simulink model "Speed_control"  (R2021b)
settings: Solver=ode1  StartTime=0.0  StopTime=inf  FixedStep=0.002  RelTol=1e-3  EnableMultiTasking=on
undefined symbols (not defined in the file or in its folder): HIL, qc_get_step_size
libraries: quarc_library x3

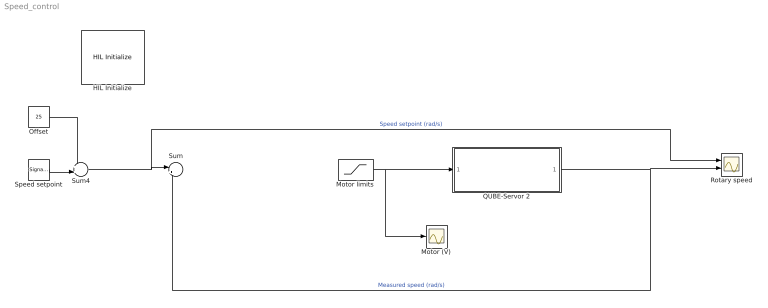
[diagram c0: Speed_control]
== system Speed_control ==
  HIL Initialize : quarc_library/Data Acquisition/Generic/Configuration/HIL Initialize  object_name=HIL-1  board_type=qube_servo2_usb  board_number=0  board_options=""  exclusive=off  active=on  hardware_clocks=[0]  clock_modes=[]  initial_clock_frequencies=[]  set_clock_params_at_start=off  set_clock_params_at_switch_in=off  set_clock_frequencies_at_start=off  set_clock_frequencies_at_switch_in=off  analog_input_channels=[0]  analog_input_configurations=[]  analog_input_maximums=3  analog_input_minimums=-3  set_analog_input_params_at_start=off  set_analog_input_params_at_switch_in=off  analog_output_channels=[0]  analog_output_maximums=15  analog_output_minimums=-15  initial_analog_outputs=[0]  final_analog_outputs=[0]  watchdog_analog_outputs=0  set_analog_output_params_at_start=off  set_analog_output_params_at_switch_in=off  set_analog_outputs_at_start=on  set_analog_outputs_at_switch_in=off  set_analog_outputs_at_terminate=on  set_analog_outputs_at_switch_out=off  set_analog_outputs_on_watchdog=on  digital_input_channels=[]  digital_output_channels=[0]  digital_output_configuration=[]  initial_digital_outputs=[1]  final_digital_outputs=[0]  watchdog_digital_outputs=[0]  set_digital_output_params_at_start=off  set_digital_output_params_at_switch_in=off  set_digital_outputs_at_start=on  set_digital_outputs_at_switch_in=off  set_digital_outputs_at_terminate=on  set_digital_outputs_at_switch_out=off  set_digital_outputs_on_watchdog=on  encoder_channels=[0:1]  quadrature=[4]  encoder_filter_frequency=[]  initial_encoder_counts=[0]  set_encoder_params_at_start=off  set_encoder_params_at_switch_in=off  set_encoder_counts_at_start=on  set_encoder_counts_at_switch_in=off  pwm_channels=[]  pwm_modes=[]  pwm_frequency=[]  pwm_configuration=[]  pwm_alignment=[]  pwm_polarity=[]  pwm_leading_deadband=[]  pwm_trailing_deadband=[]  initial_pwm_outputs=[]  final_pwm_outputs=[]  watchdog_pwm_outputs=[]  set_pwm_params_at_start=off  set_pwm_params_at_switch_in=off  set_pwm_outputs_at_start=off  set_pwm_outputs_at_switch_in=off  set_pwm_outputs_at_terminate=off  set_pwm_outputs_at_switch_out=off  set_pwm_outputs_on_watchdog=off  other_output_channels=[11000:11002]  initial_other_outputs=[0 1 0]  final_other_outputs=[1 0 0]  watchdog_other_outputs=[0 0 1]  set_other_outputs_at_start=on  set_other_outputs_at_switch_in=off  set_other_outputs_at_terminate=on  set_other_outputs_at_switch_out=off  set_other_outputs_on_watchdog=on
  Motor (V) : Scope
  Motor limits : Saturate  UpperLimit=10  LowerLimit=-10
  Offset : Constant  Value=25
  QUBE-Servor 2 : Subsystem
  Rotary speed : Scope  NumInputPorts=2
  Speed setpoint : SignalGenerator  WaveForm=square  Amplitude=5  Frequency=0.2
  Sum : Sum  Inputs=|+-
  Sum4 : Sum  Inputs=++|
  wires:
  Sum4/1 -> Rotary speed/1, Sum/1  "Speed setpoint (rad/s)"
  Speed setpoint/1 -> Sum4/2
  Offset/1 -> Sum4/1
  Sum/1 -> ?
  Motor limits/1 -> QUBE-Servor 2/1(In1), Motor (V)/1
  QUBE-Servor 2/1(measured speed (rad/s)) -> Rotary speed/2, Sum/2  "Measured speed (rad/s)"

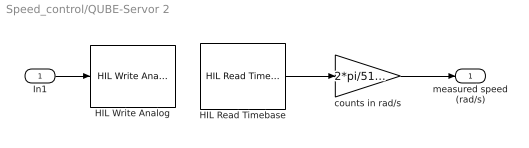
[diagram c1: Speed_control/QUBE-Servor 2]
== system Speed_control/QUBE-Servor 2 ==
  In1 : Inport
  HIL Read Timebase : quarc_library/Data Acquisition/Generic/Timebases/HIL Read Timebase  object_name=HIL-1  clock=0  analog_channels=[]  encoder_channels=[]  digital_channels=[]  other_channels=[14000]  active=on  vector_output=off  data_type_mode=Inherit via back propagation  encoder_data_type=double  digital_data_type=boolean  overflow_mode=Error on overflow  samples_in_buffer=max(ceil(1/qc_get_step_size), 1)
  HIL Write Analog : quarc_library/Data Acquisition/Generic/Immediate I//O/HIL Write Analog  object_name=HIL-1  channels=0  sample_time=-1  active=off  vector_input=off
  counts in rad/s : Gain  Gain=2*pi/512/4
  measured speed (rad/s) : Outport
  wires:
  In1/1 -> HIL Write Analog/1
  counts in rad/s/1 -> measured speed (rad/s)/1
  HIL Read Timebase/1 -> counts in rad/s/1
